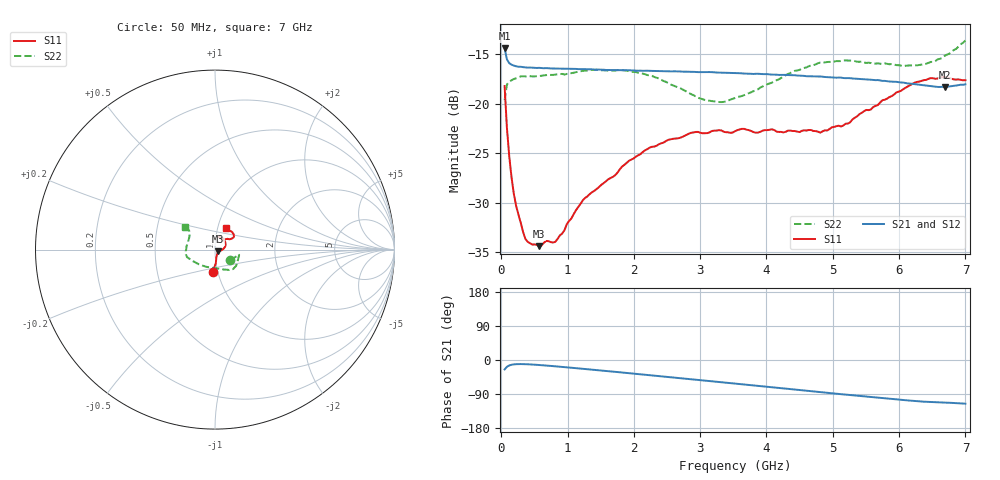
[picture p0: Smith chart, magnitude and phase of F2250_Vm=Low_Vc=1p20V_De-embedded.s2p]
! Integrated Device Technology
! Corporate Headquarters
! 6024 Silver Creek Valley Road
! San Jose, CA 95138  USA
! Phone:  1-408-284-8200
! Toll Free:  1-800-223-1366
! Webpage:  http://www.idt.com/
! Timing and RF Division
! 515 Groton Road, Suite 102
! Westford, MA 01886-6024
! Device:  F2250
! Description: Voltage Variable RF Attenuator
! Frequency:  50.0 -  6000.00 MHz
! Package:  3x3 mm Thin QFN Plastic Package: 16 pin
! Ports:  2 RF, 3 DC
!  Pin  1  = GND
!  Pin  2  = NC
!  Pin  3  = RF1  = Port 1
!  Pin  4  = NC
!  Pin  5  = GND
!  Pin  6  = GND
!  Pin  7  = GND
!  Pin  8  = GND
!  Pin  9  = NC
!  Pin 10  = RF2  = Port 2
!  Pin 11  = NC
!  Pin 12  = GND
!  Pin 13  = GND
!  Pin 14  = VCNTRL
!  Pin 15  = VDD
!  Pin 16  = VMODE
! Vcntrl:  1.200 Volts
! Vmode:  +0.000 Volts
! Vdd:  +3.30  Volts
! Current:  1.192 mA
! Data:  The device was measured on a the F2250 evaluation board which has
!  individual transmission lines to the RF pins.  Data was collected
!  using a calibrated network analyzer.  The evaluation board was
!  de-embedded using a TRL calibration technique.
!  The reference plane is the edge of the package pin.
! Misc:  SN 10
!  Action Tracker AT0258
! Date Measured:  2014-11-26
! Date:  2015-10-15  MJV
! Note:
!  Integrated Device Technology supplies this data as a sample of measured
!  data at the package pin for this product.  Your particular data for this
!  product may vary.
!  Data was taken at 25 degrees C.
!  Integrated Device Technology reserves the right to change this data at anytime.
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# GHz S dB R 50
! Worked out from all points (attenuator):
!   201 points, 50 MHz to 7 GHz, reference 50 ohm
!   highest |S21| = -14.37 dB at 50 MHz (marker M1); lowest = -18.3 dB at 6.687 GHz (marker M2)
!   lowest |S11| = -34.4 dB at 571.2 MHz (marker M3), VSWR 1.04, Z = 51.7 - j0.954 ohm
!   |S11| at or under -10 dB: start of sweep to end of sweep
!   |S22| runs from -19.8 to -13.6 dB; largest |S21 - S12| = 0.00057
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0.05  -18.19 -95.7  -14.37 -24.8  -14.37 -24.8  -19.64 -34.8
0.08475  -22.42 -86.5  -15.50 -17.9  -15.49 -17.9  -18.05 -17.3
0.1195  -25.27 -82.9  -15.87 -14.4  -15.86 -14.4  -17.75 -12.8
0.15425  -27.43 -79.4  -16.03 -12.6  -16.04 -12.6  -17.62 -11.6
0.22375  -30.32 -67.9  -16.20 -11.0  -16.19 -11.0  -17.41 -11.8
0.36275  -33.66 -50.5  -16.30 -11.0  -16.30 -11.0  -17.22 -13.1
0.57125  -34.40 -29.0  -16.35 -13.2  -16.35 -13.2  -17.19 -18.4
0.6755  -33.87 -26.9  -16.38 -14.6  -16.38 -14.6  -17.09 -21.2
0.8145  -33.96 -18.9  -16.42 -16.7  -16.42 -16.7  -17.04 -25.3
1.2315  -29.74 -9.6  -16.48 -23.3  -16.49 -23.3  -16.64 -35.5
1.9265  -25.75 9.8  -16.60 -34.7  -16.61 -34.7  -16.68 -48.0
2.37825  -24.08 21.3  -16.68 -42.3  -16.67 -42.4  -17.43 -57.5
2.86475  -22.92 36.9  -16.76 -50.8  -16.75 -50.8  -19.02 -75.2
3.0385  -22.98 43.3  -16.78 -53.8  -16.76 -53.8  -19.55 -84.5
3.3165  -22.68 52.8  -16.84 -58.6  -16.84 -58.6  -19.82 -102.5
3.525  -22.76 57.9  -16.88 -62.3  -16.88 -62.3  -19.40 -116.2
4.7065  -22.74 65.6  -17.20 -82.9  -17.20 -82.9  -16.08 -163.1
5.22775  -21.99 48.2  -17.39 -91.9  -17.38 -91.9  -15.61 -173.3
5.85325  -19.31 33.6  -17.73 -102.4  -17.73 -102.4  -15.99 172.5
6.305  -17.74 36.0  -18.07 -109.1  -18.07 -109.1  -16.06 157.1
6.68725  -17.27 46.0  -18.29 -112.4  -18.29 -112.4  -15.14 144.4
7  -17.60 63.4  -18.02 -115.3  -18.03 -115.3  -13.58 142.6
